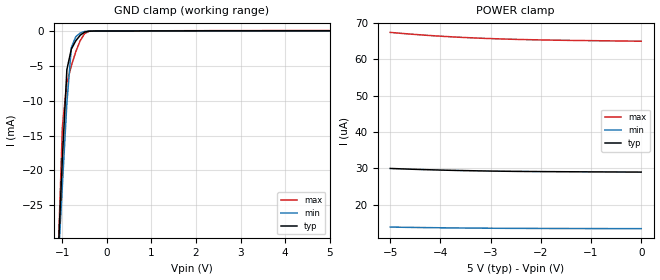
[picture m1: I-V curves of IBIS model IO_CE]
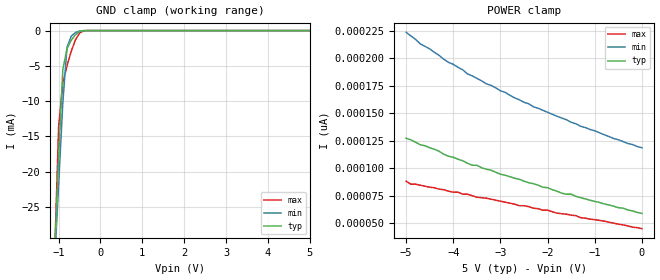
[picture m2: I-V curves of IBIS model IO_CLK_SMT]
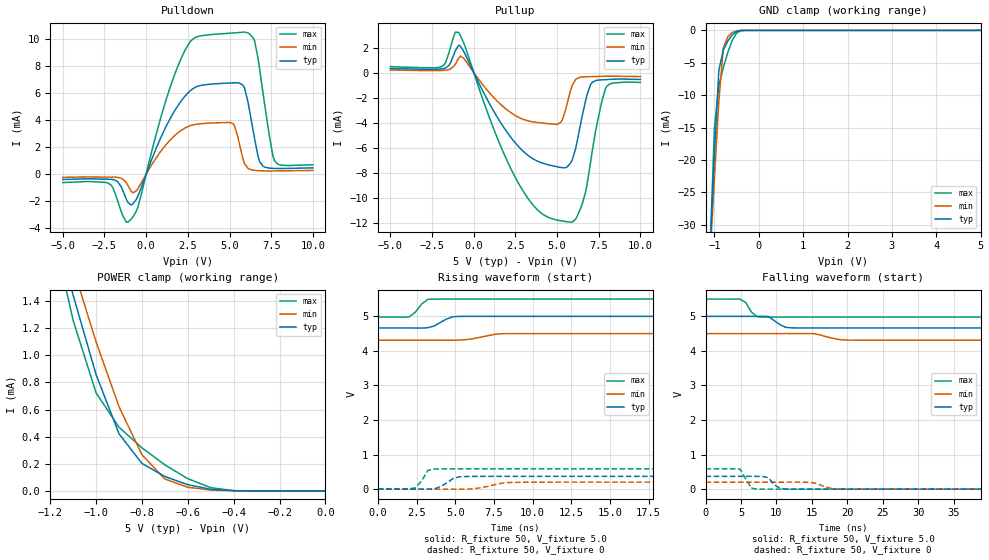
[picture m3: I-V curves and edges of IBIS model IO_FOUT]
[IBIS Ver]   3.2
[Comment Char]   |_char
[File name]   rx8803lc_5.ibs
[File Rev]   1.0
[Date]   Jan 16, 2013
[Source]   This file orginated at SEIKO EPSON Corp.
[Copyright]
   Copyright 2013, SEIKO EPSON Corp.
[Component]   8803lc_5
[Manufacturer]  SEIKO EPSON Corp.
[Package]
| variable   typ   min   max
R_pkg   55.81m   NA   NA
L_pkg   4.67nH   NA   NA
C_pkg   220.0fF   NA   NA
[Pin] signal_name   model_name
1   NC   NC
2   FOE   IO_FOE
3   VDD   POWER
4   FOUT   IO_FOUT
5   SCL   IO_CLK_SMT
6   CE   IO_CE
7   NC   NC
8   SDA   IO_DIO_SMT
9   T2(VPP)   POWER
10   VSS   GND
11   /INT   IO_IRQ
12   EVIN   IO_STAMP
| Models and submodels in the file (9): IO_CE (Input), IO_CLK_SMT (Input), IO_FOUT (3-state), IO_TEST (Input), IO_FOE (Input), IO_STAMP (Input), IO_IRQ (Open_drain), IO_DIO_SMT (I/O_open_drain), IO_IN (Input)
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[Model]   IO_CE
Model_type Input
Enable Active-Low
Polarity Non-Inverting
Vinh=4.0
Vinl=1.0
C_comp   5p   4p   6p
[Temperature Range] 25   85   -40
[Voltage Range]   5.0   4.5   5.5
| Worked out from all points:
|   GND clamp passes 1 mA (typ) near -0.65 V on its own axis
[GND Clamp]
-5V       -651.7mA   -534.8mA   -828.6mA
-1.1V     -32.77mA   -33.87mA   -32.85mA
-1V       -18.1mA    -22.01mA   -13.66mA
-900mV    -5.535mA   -10.31mA   -7.453mA
-800mV    -2.591mA   -2.383mA   -4.992mA
-700mV    -1.404mA   -815.4uA   -2.967mA
-600mV    -601.6uA   -287.5uA   -1.367mA
-500mV    -153uA     -66.42uA   -360.1uA
-400mV    -21.86uA   -10.85uA   -41.85uA
-300mV    -5.712uA   -3.176uA   -10.59uA
5V        28.94uA    13.37uA    64.9uA
[POWER Clamp]
-5V       29.94uA    13.79uA    67.42uA
-4.8V     29.84uA    13.75uA    67.18uA
-4.5V     29.7uA     13.69uA    66.84uA
-4.3V     29.61uA    13.65uA    66.64uA
-4V       29.5uA     13.6uA     66.37uA
-3.8V     29.43uA    13.57uA    66.21uA
-3.5V     29.34uA    13.53uA    66uA
-3V       29.22uA    13.48uA    65.71uA
-2.5V     29.14uA    13.44uA    65.5uA
-1.9V     29.07uA    13.41uA    65.32uA
-1.2V     29.01uA    13.39uA    65.18uA
0V        28.94uA    13.36uA    64.99uA
[Model]   IO_CLK_SMT
Model_type Input
Enable Active-Low
Polarity Non-Inverting
Vinh=4.0
Vinl=1.0
C_comp   5p   4p   6p
[Temperature Range] 25   85   -40
[Voltage Range]   5.0   4.5   5.5
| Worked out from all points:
|   GND clamp passes 1 mA (typ) near -0.65 V on its own axis
[GND Clamp]
-5V       -640.1mA   -524.9mA   -814.3mA
-1.1V     -32.43mA   -33.46mA   -32.61mA
-1V       -17.96mA   -21.79mA   -13.59mA
-900mV    -5.499mA   -10.22mA   -7.421mA
-800mV    -2.576mA   -2.362mA   -4.965mA
-700mV    -1.392mA   -807.3uA   -2.943mA
-600mV    -591.5uA   -281.9uA   -1.347mA
-500mV    -144.6uA   -61.93uA   -343.6uA
-400mV    -15.25uA   -7.313uA   -28.72uA
-300mV    -812.1nA   -557.3nA   -822.7nA
5V        58.89pA    126pA      40.93pA
[POWER Clamp]
-5V       127.3pA    223.7pA    88.22pA
-4.9V     126pA      220.6pA    85.49pA
-4.7V     121.4pA    213.3pA    84.58pA
-4.4V     117.3pA    205.5pA    82.31pA
-4.2V     112.8pA    199.2pA    80.49pA
-3.8V     106.9pA    189.6pA    76.4pA
-3.7V     104.6pA    186pA      76.4pA
-2.7V     90.95pA    164.2pA    67.3pA
-1.7V     77.31pA    145.7pA    58.66pA
-1.5V     76.4pA     141.9pA    57.3pA
-1.3V     73.21pA    138.2pA    55.02pA
0V        58.89pA    118.7pA    45.02pA
[Model]   IO_FOUT
Model_type 3-state
Enable Active-High
Polarity Non-Inverting
Vmeas=2.50
C_comp   5p   4p   6p
[Temperature Range] 25   85   -40
[Voltage Range]   5.0   4.5   5.5
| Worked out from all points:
|   slope of the pulldown table from 0 to 0.75 V, typ, clamps not added: 321 ohm
|   slope of the pullup table from 0 to 0.75 V, typ, clamps not added: 374 ohm
|   GND clamp passes 1 mA (typ) near -0.63 V on its own axis
|   POWER clamp passes 1 mA (typ) near -1.02 V on its own axis
|   falling waveform, R_fixture 50, V_fixture 5.0: 20-80 % time 1.49ns typ, 2.16ns min, 1.04ns max; typ from 5 V to 4.66 V
|   falling waveform, R_fixture 50, V_fixture 0: 20-80 % time 1.11ns typ, 1.79ns min, 1.04ns max; typ from 0.371 V to 0 V
|   rising waveform, R_fixture 50, V_fixture 5.0: 20-80 % time 819ps typ, 1.28ns min, 637ps max; typ from 4.66 V to 5 V
|   rising waveform, R_fixture 50, V_fixture 0: 20-80 % time 768ps typ, 1.27ns min, 557ps max; typ from 0 V to 0.371 V
[Pullup]
-5V       329.6uA    205.5uA    474.4uA
-2V       287.7uA    169.6uA    448.8uA
-900mV    2.189mA    1.173mA    3.197mA
1.4V      -3.541mA   -2.268mA   -5.182mA
2.9V      -6.197mA   -3.698mA   -9.332mA
4.1V      -7.217mA   -4.025mA   -11.27mA
5.2V      -7.57mA    -3.994mA   -11.83mA
5.8V      -7.233mA   -1.458mA   -11.94mA
6.5V      -3.485mA   -348.8uA   -10.51mA
7V        -966.5uA   -325.2uA   -7.212mA
7.9V      -564.2uA   -289.6uA   -1.275mA
10V       -549.9uA   -317.8uA   -785.4uA
[Pulldown]
-5V       -390.6uA   -232.1uA   -617.2uA
-2.3V     -364.7uA   -211.4uA   -640.6uA
-1.1V     -2.068mA   -811.8uA   -3.543mA
-500mV    -1.636mA   -1.074mA   -2.448mA
1.2V      3.536mA    2.193mA    5.51mA
2.6V      6.113mA    3.563mA    9.719mA
5.2V      6.747mA    3.745mA    10.43mA
5.9V      6.372mA    780.5uA    10.5mA
6.5V      2.656mA    283.8uA    9.872mA
6.8V      947.8uA    259.7uA    7.82mA
7.7V      428.1uA    245.5uA    995.5uA
10V       470.7uA    280.4uA    699.2uA
[GND Clamp]
-5V       -673.6mA   -553.9mA   -855.1mA
-1.1V     -34.07mA   -35.2mA    -34.52mA
-1V       -19.07mA   -22.99mA   -15.1mA
-900mV    -6.217mA   -10.96mA   -8.569mA
-800mV    -3.038mA   -2.745mA   -5.779mA
-700mV    -1.663mA   -981.4uA   -3.456mA
-600mV    -716.1uA   -347.4uA   -1.603mA
-500mV    -178.4uA   -77.34uA   -418.8uA
-400mV    -19.08uA   -9.208uA   -35.91uA
-300mV    -1.02uA    -704.8nA   -1.036uA
5V        101.9pA    6.525uA    74.12pA
[POWER Clamp]
-5V       33.51mA    29.11mA    40.73mA
-1.2V     2.101mA    2.224mA    2.001mA
-1.1V     1.442mA    1.642mA    1.256mA
-1V       856.8uA    1.098mA    722.6uA
-900mV    420.7uA    620.6uA    469.5uA
-800mV    202.7uA    266uA      317.8uA
-700mV    106.2uA    87.94uA    192.1uA
-600mV    46.01uA    26.93uA    90.33uA
-500mV    12.08uA    6.525uA    23.88uA
-400mV    1.581uA    1.101uA    2.09uA
0V        101.9pA    182.1pA    86.4pA
[Falling Waveform]
R_fixture=50
V_fixture=5.0
V_fixture_min=4.5
V_fixture_max=5.5
0s        5V         4.5V       5.5V
4.848ns   5V         4.5V       5.5V
5.657ns   5V         4.5V       5.404V
6.465ns   5V         4.5V       5.127V
7.273ns   5V         4.5V       4.987V
8.081ns   5V         4.5V       4.981V
12.12ns   4.668V     4.5V       4.979V
15.35ns   4.664V     4.498V     4.979V
20.2ns    4.664V     4.314V     4.979V
80ns      4.664V     4.31V      4.979V
[Falling Waveform]
R_fixture=50
V_fixture=0
V_fixture_min=0
V_fixture_max=0
0s        370.7mV    202.7mV    587.3mV
4.848ns   370.7mV    202.7mV    581.1mV
6.465ns   371.4mV    202.7mV    31.52mV
7.273ns   371.5mV    202.7mV    -30.96uV
8.889ns   326.8mV    202.8mV    7.983uV
9.697ns   126.1mV    202.9mV    2.49uV
11.31ns   1.001mV    203.2mV    -6.219uV
15.35ns   1.403uV    180mV      -5.148uV
19.39ns   -8.753uV   250.9uV    -4.489uV
80ns      7.818uV    -11.01uV   -1.596uV
[Rising Waveform]
R_fixture=50
V_fixture=5.0
V_fixture_min=4.5
V_fixture_max=5.5
0s        4.664V     4.31V      4.979V
2.02ns    4.664V     4.31V      4.985V
2.424ns   4.662V     4.31V      5.123V
2.828ns   4.66V      4.31V      5.356V
3.232ns   4.672V     4.31V      5.493V
3.636ns   4.719V     4.31V      5.499V
4.444ns   4.924V     4.307V     5.5V
5.253ns   4.999V     4.314V     5.5V
8.081ns   5V         4.498V     5.5V
40ns      5V         4.5V       5.5V
[Rising Waveform]
R_fixture=50
V_fixture=0
V_fixture_min=0
V_fixture_max=0
0s        0V         0V         0V
2.424ns   71.13uV    -2.792uV   42.01mV
2.828ns   36.63uV    -1.002uV   239.3mV
3.232ns   -677.3uV   4.637uV    542.2mV
4.04ns    69.36mV    66.92uV    586.4mV
4.848ns   303.4mV    -47.72uV   587.1mV
6.061ns   368.9mV    4.211mV    587.3mV
8.081ns   370.6mV    177.5mV    587.3mV
9.293ns   370.7mV    199.2mV    587.3mV
40ns      370.7mV    202.7mV    587.3mV
[Ramp]
R_load=50
dV/dt_r   2.224E-1/7.538E-10   1.216E-1/1.220E-9   3.524E-1/4.631E-10
dV/dt_f   2.014E-1/1.343E-9   1.139E-1/2.129E-9   3.123E-1/9.046E-10
|[End   IO_FOUT
